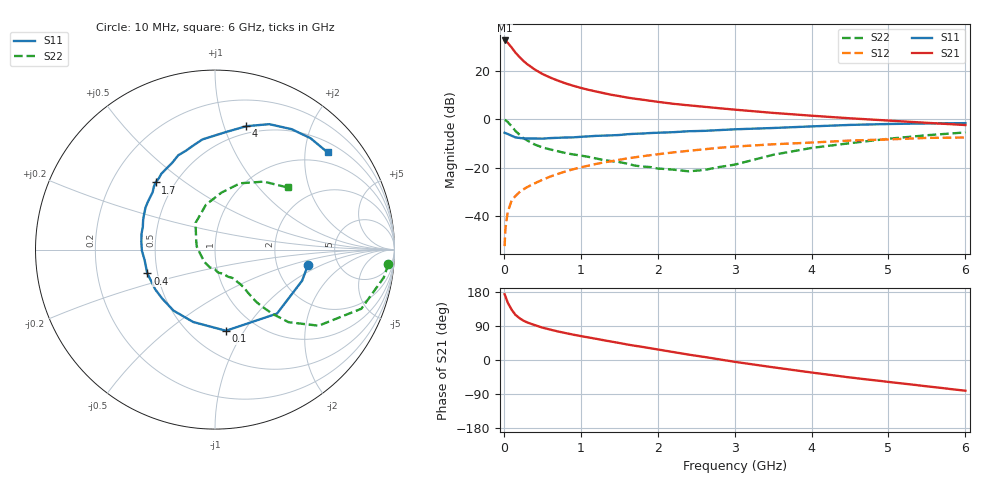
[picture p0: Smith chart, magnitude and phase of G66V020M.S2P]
! SIEMENS Small Signal Semiconductors
! BFG193
! Si NPN RF Bipolar Junction Transistor in SOT223
! VCE = 6 V  IC = 20 mA
! Common Emitter S-Parameters:  August  1996
# GHz  S  MA  R  50
!  f  S11  S21  S12  S22
! GHz  MAG  ANG  MAG  ANG  MAG  ANG  MAG  ANG
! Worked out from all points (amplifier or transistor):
!   36 points, 10 MHz to 6 GHz, reference 50 ohm
!   highest |S21| = 32.5 dB at 10 MHz (marker M1)
!   |S21| within 3 dB of that: start of sweep to 103.2 MHz
!   unconditionally stable (mu >= 1): 722.5 MHz to 2.438 GHz
!   at 250 MHz: K = 0.73, MSG = 26.6 dB, |S12| = -29.0 dB
!   at 1.4 GHz: K = 1.05, MAG = 12.3 dB, |S12| = -17.3 dB
!   at 6 GHz: K = 0.88, MSG = 2.6 dB, |S12| = -7.6 dB
!   S11 on the Smith chart (normalised r, x): 10 MHz: 3.01, -0.73; 100 MHz: 0.73, -0.83; 400 MHz: 0.44, -0.14; 1.7 GHz: 0.39, +0.39; 4 GHz: 0.43, +1.19; 6 GHz: 0.72, +2.51
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0.01  0.5243 -9.6  42.09 173.5  0.0024 92.3  0.9692 -4.7
0.02  0.5155 -19.6  41.49 168.3  0.0054 86.2  0.9531 -9.4
0.05  0.4964 -45.9  37.8 151.7  0.0121 73.8  0.8795 -22.0
0.1  0.4562 -82.3  30.26 133.2  0.0209 64.2  0.7162 -36.3
0.15  0.4213 -106.7  23.73 119.3  0.0259 59.0  0.5762 -44.6
0.2  0.4111 -124.2  19.41 111.0  0.0309 59.2  0.484 -48.0
0.25  0.4013 -137.0  16.15 104.4  0.0353 58.6  0.4116 -50.5
0.3  0.4 -146.4  13.81 99.4  0.0394 59.4  0.3671 -51.8
0.4  0.3997 -160.6  10.66 92.2  0.0474 60.1  0.3011 -52.6
0.5  0.3966 -171.6  8.602 85.5  0.0561 60.6  0.2622 -52.8
0.6  0.4071 -179.0  7.263 80.4  0.0651 60.8  0.2383 -53.8
0.7  0.4128 174.1  6.275 75.5  0.0741 60.2  0.2185 -55.3
0.9  0.4216 162.5  4.902 67.0  0.0926 58.1  0.1877 -57.9
1.1  0.4419 153.3  4.038 59.5  0.11 55.6  0.1669 -64.7
1.4  0.4643 141.2  3.179 48.5  0.1362 50.6  0.1361 -75.5
1.7  0.4995 131.5  2.647 37.7  0.1631 45.2  0.1106 -89.5
2.2  0.5389 116.3  2.08 21.0  0.2062 34.6  0.0911 -130.0
3.5  0.6578 84.7  1.348 -19.2  0.3034 4.8  0.184 126.1
4  0.7097 75.7  1.18 -33.0  0.3294 -4.8  0.255 101.4
4.5  0.7615 66.6  1.043 -46.1  0.362 -14.9  0.3198 83.5
5.5  0.8175 49.4  0.841 -69.4  0.4112 -38.4  0.4664 54.3
6  0.8287 40.8  0.757 -81.1  0.4184 -52.1  0.5329 40.5
